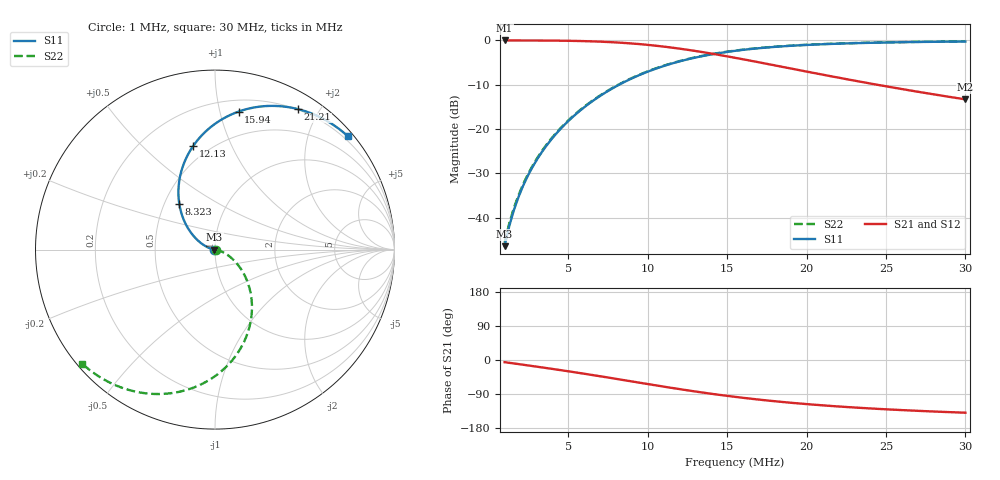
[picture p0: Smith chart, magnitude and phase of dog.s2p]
# MHz S RI R 50.0
!SimSmith 16.10a
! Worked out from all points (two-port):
!   100 points, 1 MHz to 30 MHz, reference 50 ohm
!   highest |S21| = 0.00 dB at 1 MHz (marker M1); lowest = -13.3 dB at 30 MHz (marker M2)
!   |S21| within 3 dB of the highest: start of sweep to 14.07 MHz
!   lowest |S11| = -46.4 dB at 1 MHz (marker M3), VSWR 1.01, Z = 49.5 + j0.0503 ohm
!   |S11| at or under -10 dB: start of sweep to 8.204 MHz
!   |S22| runs from -45.6 to -0.2 dB; largest |S21 - S12| = 0
!   S11 on the Smith chart (normalised r, x): 1 MHz: 0.99, +0.00; 8.323 MHz: 0.59, +0.34; 12.13 MHz: 0.41, +0.72; 15.94 MHz: 0.29, +1.14; 21.21 MHz: 0.19, +1.74; 30 MHz: 0.12, +2.70
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1  -0.00475 0.000508  0.9947 -0.1  0.9947 -0.1  0.00519 -0.000547
1.292929  -0.00799 0.00109  0.9912 -0.1292  0.9912 -0.1292  0.00857 -0.00116
1.585859  -0.012 0.00201  0.9868 -0.1585  0.9868 -0.1585  0.0128 -0.00211
1.878788  -0.0169 0.00333  0.9815 -0.1877  0.9815 -0.1877  0.0177 -0.00348
2.171717  -0.0225 0.00514  0.9753 -0.2169  0.9753 -0.2169  0.0234 -0.00534
2.757576  -0.0358 0.0105  0.9598 -0.2751  0.9598 -0.2751  0.037 -0.0108
3.343434  -0.0517 0.0187  0.9403 -0.333  0.9403 -0.333  0.0532 -0.0191
4.222222  -0.0794 0.0373  0.9026 -0.4183  0.9026 -0.4183  0.0811 -0.0381
5.979798  -0.1404 0.1034  0.7944 -0.5782  0.7944 -0.5782  0.1425 -0.1049
7.151515  -0.1762 0.1711  0.6972 -0.6695  0.6972 -0.6695  0.1785 -0.1732
8.323232  -0.1992 0.2563  0.5824 -0.7408  0.5824 -0.7408  0.2014 -0.2591
9.494949  -0.2025 0.3539  0.4558 -0.7862  0.4558 -0.7862  0.2045 -0.3572
10.66667  -0.1819 0.4557  0.3256 -0.8026  0.3256 -0.8026  0.1836 -0.4595
12.13131  -0.1231 0.5753  0.1722 -0.7837  0.1722 -0.7837  0.1241 -0.5795
13.88889  -0.0156 0.6891  0.0202 -0.7167  0.0202 -0.7167  0.0158 -0.6936
15.64646  0.1108 0.7612  -0.0873 -0.6242  -0.0873 -0.6242  -0.1113 -0.7656
15.93939  0.1322 0.7693  -0.101 -0.6079  -0.101 -0.6079  -0.1328 -0.7737
17.9899  0.276 0.7992  -0.1683 -0.4961  -0.1683 -0.4961  -0.2773 -0.8032
20.62626  0.4325 0.7894  -0.2017 -0.373  -0.2017 -0.373  -0.4343 -0.7929
21.21212  0.4622 0.7827  -0.2039 -0.3498  -0.2039 -0.3498  -0.4641 -0.7861
25.31313  0.6244 0.7165  -0.194 -0.2251  -0.194 -0.2251  -0.6266 -0.7191
30  0.7387 0.6328  -0.1636 -0.1417  -0.1636 -0.1417  -0.7409 -0.6347
